| TEXAS INSTRUMENTS INCORPORATED
| Standard Linear and Logic Group
| IBIS Model of SN74AVC32T245
| 32-Bit Dual-Supply Bus Transeiver with Configurable Voltage Translation and
| 3-State Outputs
| This file contains package information for the following:
|  LFBGA 96-pin (GKE)  package as [Component] AVC32T245_GKE
|  LFBGA 96-pin (ZKE)  package as [Component] AVC32T245_ZKE
| This device can be powered at the following Vccs:
|  1.2 volt Vcc
|  1.5 volt Vcc
|  1.8 volt Vcc
|  2.5 volt Vcc
|  3.3 volt Vcc
| This file provides unique models under the [Model Selector] for each Vcc.
| For operation at a specific Vcc, select the appropriate model after each
| [Model Selector] keyword.
[IBIS Ver]   3.2
[Comment char]  |_char
[File Name]   sn74avc32t245.ibs
[File Rev]   1.1 | x_die
[Date]   July 17, 2004
[Source]   Data created from TI-SPICE simulations at TI-SLL.
[Notes]   The following is an IBIS list for the AVC32T245.
   Please contact sllibis@ti.com with questions and
   comments concerning SLL IBIS models.
   - FILE REV HISTORY
   - 1.1 Release IBIS file on 07/17/04
   - This IBIS model was created from the AVC16T245
   - Power clamp data deleted as there is no power-clamp diode.
   - Due to the fact that the Device is 4.6-V Input/Output
   tolarent, the I/O models has some Non-Monotonic Warnings.
[Disclaimer] Property of Texas Instruments Incorporated.  Unauthorized
   reproduction and/or distribution is strictly prohibited.
   This product is protected under copyright law.
   Created  2003, (C) Copyright  2003, Texas Instruments
   Incorporated, All Rights Reserved
   UNLESS THERE IS A SIGNED, WRITTEN AGREEMENT TO THE
   CONTRARY, TEXAS INSTRUMENTS (TI) IS PROVIDING THE IBIS
   MODELS  AND WITHOUT ANY WARRANTY, EXPRESSED OR
   IMPLIED.  TI assumes no liability for:
   1) the accuracy of the IBIS models provided to your
   company;
   2) the proper functioning of these IBIS Models in your
   design or for any resulting applications; or
   3) infringement of patents, copyrights or intellectual
   property rights resulting from your use of these IBIS
   models.
   TI provides IBIS Models as a service to our customers.
   You and your company shall not distribute, sell or give
   these models to anyone else without prior written
   permission from TI.
   TI reserves the right to make changes to our products or
   to discontinue any semiconductor product or service
   without notice, and advises our customers to obtain the
   latest version of relevant information to verify, before
   placing orders, that the information being relied on is
   current.
   Please be aware that your receipt and use of the IBIS
   information provided shall serve as acceptance of these
   terms and conditions.  If you do not accept these terms,
   you should return or destroy the IBIS models and any
   other accompanying information immediately.
| Component AVC32T245_GKE 96-pin LFBGA
[Component]   AVC32T245_GKE
[Manufacturer]  Texas Instruments, Inc.
[Package]
|   typ   min   max
R_pkg   6.700e-02   5.600e-02   8.700e-02
L_pkg   2.067e-09   1.596e-09   2.867e-09
C_pkg   1.810e-13   1.460e-13   2.440e-13
[Pin]   signal_name   model_name   R_pin   L_pin   C_pin
A3   1DIR   AVC32T245_DIR   8.400e-02   2.866e-09   2.140e-13
A2   1B1   AVC32T245_IO   5.600e-02   1.650e-09   1.470e-13
A1   1B2   AVC32T245_IO   5.900e-02   1.761e-09   1.550e-13
B3   GND   GND   8.300e-02   2.828e-09   2.340e-13
B2   1B3   AVC32T245_IO   6.000e-02   1.737e-09   1.570e-13
B1   1B4   AVC32T245_IO   6.100e-02   1.767e-09   1.580e-13
C3   VCCB   POWER   8.100e-02   2.750e-09   2.280e-13
C2   1B5   AVC32T245_IO   5.700e-02   1.664e-09   1.540e-13
C1   1B6   AVC32T245_IO   6.100e-02   1.746e-09   1.620e-13
D3   GND   GND   7.900e-02   2.660e-09   2.390e-13
D2   1B7   AVC32T245_IO   5.600e-02   1.619e-09   1.520e-13
D1   1B8   AVC32T245_IO   6.100e-02   1.703e-09   1.510e-13
E2   2B1   AVC32T245_IO   6.400e-02   1.911e-09   1.680e-13
E1   2B2   AVC32T245_IO   6.100e-02   1.732e-09   1.540e-13
E3   GND   GND   7.900e-02   2.626e-09   2.290e-13
F2   2B3   AVC32T245_IO   6.400e-02   1.862e-09   1.750e-13
F1   2B4   AVC32T245_IO   6.100e-02   1.697e-09   1.520e-13
F3   VCCB   POWER   8.000e-02   2.671e-09   2.320e-13
G2   2B5   AVC32T245_IO   6.500e-02   1.908e-09   1.770e-13
G1   2B6   AVC32T245_IO   6.100e-02   1.682e-09   1.510e-13
G3   GND   GND   8.000e-02   2.678e-09   2.150e-13
H1   2B8   AVC32T245_IO   6.100e-02   1.720e-09   1.590e-13
H2   2B7   AVC32T245_IO   5.600e-02   1.596e-09   1.500e-13
H3   2DIR   AVC32T245_DIR   8.600e-02   2.851e-09   2.440e-13
J3   3DIR   AVC32T245_DIR   8.700e-02   2.852e-09   2.440e-13
J2   3B1   AVC32T245_IO   5.600e-02   1.596e-09   1.500e-13
J1   3B2   AVC32T245_IO   6.200e-02   1.721e-09   1.580e-13
K3   GND   GND   8.000e-02   2.678e-09   2.170e-13
K2   3B3   AVC32T245_IO   6.200e-02   1.741e-09   1.560e-13
K1   3B4   AVC32T245_IO   6.000e-02   1.696e-09   1.580e-13
L3   VCCB   POWER   8.000e-02   2.675e-09   2.200e-13
L2   3B5   AVC32T245_IO   6.100e-02   1.754e-09   1.570e-13
L1   3B6   AVC32T245_IO   6.100e-02   1.702e-09   1.610e-13
M3   GND   GND   7.800e-02   2.628e-09   2.210e-13
M2   3B7   AVC32T245_IO   6.200e-02   1.791e-09   1.580e-13
M1   3B8   AVC32T245_IO   6.100e-02   1.748e-09   1.570e-13
N2   4B1   AVC32T245_IO   6.200e-02   1.762e-09   1.560e-13
N1   4B2   AVC32T245_IO   7.500e-02   2.597e-09   2.180e-13
N3   GND   GND   5.900e-02   1.680e-09   1.610e-13
P2   4B3   AVC32T245_IO   6.200e-02   1.805e-09   1.660e-13
P1   4B4   AVC32T245_IO   5.700e-02   1.661e-09   1.530e-13
P3   VCCB   POWER   8.100e-02   2.751e-09   2.270e-13
R2   4B5   AVC32T245_IO   6.200e-02   1.838e-09   1.630e-13
R1   4B6   AVC32T245_IO   6.300e-02   1.845e-09   1.650e-13
R3   GND   GND   8.300e-02   2.828e-09   2.330e-13
T1   4B7   AVC32T245_IO   6.000e-02   1.754e-09   1.550e-13
T2   4B8   AVC32T245_IO   5.600e-02   1.659e-09   1.480e-13
T3   4DIR   AVC32T245_DIR   8.500e-02   2.867e-09   2.160e-13
T4   4NOE   AVC32T245_NOE   8.400e-02   2.866e-09   2.160e-13
T5   4A8   AVC32T245_IO   5.600e-02   1.658e-09   1.480e-13
T6   4A7   AVC32T245_IO   6.000e-02   1.753e-09   1.550e-13
R4   GND   GND   8.300e-02   2.828e-09   2.320e-13
R6   4A6   AVC32T245_IO   5.900e-02   1.707e-09   1.550e-13
R5   4A5   AVC32T245_IO   6.300e-02   1.838e-09   1.640e-13
P4   VCCA   POWER   8.100e-02   2.751e-09   2.270e-13
P6   4A4   AVC32T245_IO   5.700e-02   1.661e-09   1.530e-13
P5   4A3   AVC32T245_IO   6.500e-02   1.946e-09   1.760e-13
N4   GND   GND   8.200e-02   2.804e-09   2.370e-13
N6   4A2   AVC32T245_IO   5.600e-02   1.616e-09   1.500e-13
N5   4A1   AVC32T245_IO   6.200e-02   1.762e-09   1.550e-13
M6   3A8   AVC32T245_IO   6.100e-02   1.748e-09   1.570e-13
M5   3A7   AVC32T245_IO   6.200e-02   1.791e-09   1.580e-13
M4   GND   GND   7.800e-02   2.628e-09   2.210e-13
L6   3A6   AVC32T245_IO   6.000e-02   1.678e-09   1.590e-13
L5   3A5   AVC32T245_IO   6.200e-02   1.755e-09   1.570e-13
L4   VCCA   POWER   8.000e-02   2.674e-09   2.200e-13
K6   3A4   AVC32T245_IO   6.000e-02   1.673e-09   1.560e-13
K5   3A3   AVC32T245_IO   6.100e-02   1.739e-09   1.560e-13
K4   GND   GND   8.000e-02   2.677e-09   2.170e-13
J6   3A2   AVC32T245_IO   6.100e-02   1.720e-09   1.590e-13
J5   3A1   AVC32T245_IO   5.600e-02   1.596e-09   1.500e-13
J4   3NOE   AVC32T245_NOE   8.700e-02   2.852e-09   2.440e-13
H4   2NOE   AVC32T245_NOE   8.700e-02   2.852e-09   2.440e-13
H5   2A7   AVC32T245_IO   5.600e-02   1.596e-09   1.500e-13
H6   2A8   AVC32T245_IO   6.100e-02   1.720e-09   1.590e-13
G4   GND   GND   8.200e-02   2.793e-09   2.220e-13
G5   2A5   AVC32T245_IO   6.100e-02   1.682e-09   1.510e-13
G6   2A6   AVC32T245_IO   6.400e-02   1.907e-09   1.770e-13
F4   VCCA   POWER   8.000e-02   2.670e-09   2.330e-13
F6   2A4   AVC32T245_IO   6.100e-02   1.697e-09   1.520e-13
F5   2A3   AVC32T245_IO   6.400e-02   1.862e-09   1.750e-13
E4   GND   GND   7.800e-02   2.626e-09   2.300e-13
E6   2A2   AVC32T245_IO   6.100e-02   1.714e-09   1.530e-13
E5   2A1   AVC32T245_IO   6.400e-02   1.911e-09   1.680e-13
D6   1A8   AVC32T245_IO   6.100e-02   1.736e-09   1.530e-13
D5   1A7   AVC32T245_IO   5.600e-02   1.619e-09   1.520e-13
D4   GND   GND   7.900e-02   2.660e-09   2.400e-13
C6   1A6   AVC32T245_IO   5.800e-02   1.629e-09   1.550e-13
C5   1A5   AVC32T245_IO   5.700e-02   1.664e-09   1.540e-13
C4   VCCA   POWER   8.100e-02   2.750e-09   2.280e-13
B6   1A4   AVC32T245_IO   5.900e-02   1.667e-09   1.520e-13
B5   1A3   AVC32T245_IO   5.900e-02   1.736e-09   1.570e-13
B4   GND   GND   8.300e-02   2.827e-09   2.340e-13
A6   1A2   AVC32T245_IO   5.700e-02   1.610e-09   1.460e-13
A5   1A1   AVC32T245_IO   5.600e-02   1.649e-09   1.470e-13
A4   1NOE   AVC32T245_NOE   8.500e-02   2.867e-09   2.140e-13
| Component AVC32T245_ZKE 96-pin LFBGA
[Component]   AVC32T245_ZKE
[Manufacturer]  Texas Instruments, Inc.
[Package]
|   typ   min   max
R_pkg   6.700e-02   5.600e-02   8.700e-02
L_pkg   2.067e-09   1.596e-09   2.867e-09
C_pkg   1.810e-13   1.460e-13   2.440e-13
[Pin]   signal_name   model_name   R_pin   L_pin   C_pin
A3   1DIR   AVC32T245_DIR   8.400e-02   2.866e-09   2.140e-13
A2   1B1   AVC32T245_IO   5.600e-02   1.650e-09   1.470e-13
A1   1B2   AVC32T245_IO   5.900e-02   1.761e-09   1.550e-13
B3   GND   GND   8.300e-02   2.828e-09   2.340e-13
B2   1B3   AVC32T245_IO   6.000e-02   1.737e-09   1.570e-13
B1   1B4   AVC32T245_IO   6.100e-02   1.767e-09   1.580e-13
C3   VCCB   POWER   8.100e-02   2.750e-09   2.280e-13
C2   1B5   AVC32T245_IO   5.700e-02   1.664e-09   1.540e-13
C1   1B6   AVC32T245_IO   6.100e-02   1.746e-09   1.620e-13
D3   GND   GND   7.900e-02   2.660e-09   2.390e-13
D2   1B7   AVC32T245_IO   5.600e-02   1.619e-09   1.520e-13
D1   1B8   AVC32T245_IO   6.100e-02   1.703e-09   1.510e-13
E2   2B1   AVC32T245_IO   6.400e-02   1.911e-09   1.680e-13
E1   2B2   AVC32T245_IO   6.100e-02   1.732e-09   1.540e-13
E3   GND   GND   7.900e-02   2.626e-09   2.290e-13
F2   2B3   AVC32T245_IO   6.400e-02   1.862e-09   1.750e-13
F1   2B4   AVC32T245_IO   6.100e-02   1.697e-09   1.520e-13
F3   VCCB   POWER   8.000e-02   2.671e-09   2.320e-13
G2   2B5   AVC32T245_IO   6.500e-02   1.908e-09   1.770e-13
G1   2B6   AVC32T245_IO   6.100e-02   1.682e-09   1.510e-13
G3   GND   GND   8.000e-02   2.678e-09   2.150e-13
H1   2B8   AVC32T245_IO   6.100e-02   1.720e-09   1.590e-13
H2   2B7   AVC32T245_IO   5.600e-02   1.596e-09   1.500e-13
H3   2DIR   AVC32T245_DIR   8.600e-02   2.851e-09   2.440e-13
J3   3DIR   AVC32T245_DIR   8.700e-02   2.852e-09   2.440e-13
J2   3B1   AVC32T245_IO   5.600e-02   1.596e-09   1.500e-13
J1   3B2   AVC32T245_IO   6.200e-02   1.721e-09   1.580e-13
K3   GND   GND   8.000e-02   2.678e-09   2.170e-13
K2   3B3   AVC32T245_IO   6.200e-02   1.741e-09   1.560e-13
K1   3B4   AVC32T245_IO   6.000e-02   1.696e-09   1.580e-13
L3   VCCB   POWER   8.000e-02   2.675e-09   2.200e-13
L2   3B5   AVC32T245_IO   6.100e-02   1.754e-09   1.570e-13
L1   3B6   AVC32T245_IO   6.100e-02   1.702e-09   1.610e-13
M3   GND   GND   7.800e-02   2.628e-09   2.210e-13
M2   3B7   AVC32T245_IO   6.200e-02   1.791e-09   1.580e-13
M1   3B8   AVC32T245_IO   6.100e-02   1.748e-09   1.570e-13
N2   4B1   AVC32T245_IO   6.200e-02   1.762e-09   1.560e-13
N1   4B2   AVC32T245_IO   7.500e-02   2.597e-09   2.180e-13
N3   GND   GND   5.900e-02   1.680e-09   1.610e-13
P2   4B3   AVC32T245_IO   6.200e-02   1.805e-09   1.660e-13
P1   4B4   AVC32T245_IO   5.700e-02   1.661e-09   1.530e-13
P3   VCCB   POWER   8.100e-02   2.751e-09   2.270e-13
R2   4B5   AVC32T245_IO   6.200e-02   1.838e-09   1.630e-13
R1   4B6   AVC32T245_IO   6.300e-02   1.845e-09   1.650e-13
R3   GND   GND   8.300e-02   2.828e-09   2.330e-13
T1   4B7   AVC32T245_IO   6.000e-02   1.754e-09   1.550e-13
T2   4B8   AVC32T245_IO   5.600e-02   1.659e-09   1.480e-13
T3   4DIR   AVC32T245_DIR   8.500e-02   2.867e-09   2.160e-13
T4   4NOE   AVC32T245_NOE   8.400e-02   2.866e-09   2.160e-13
T5   4A8   AVC32T245_IO   5.600e-02   1.658e-09   1.480e-13
T6   4A7   AVC32T245_IO   6.000e-02   1.753e-09   1.550e-13
R4   GND   GND   8.300e-02   2.828e-09   2.320e-13
R6   4A6   AVC32T245_IO   5.900e-02   1.707e-09   1.550e-13
R5   4A5   AVC32T245_IO   6.300e-02   1.838e-09   1.640e-13
P4   VCCA   POWER   8.100e-02   2.751e-09   2.270e-13
P6   4A4   AVC32T245_IO   5.700e-02   1.661e-09   1.530e-13
P5   4A3   AVC32T245_IO   6.500e-02   1.946e-09   1.760e-13
N4   GND   GND   8.200e-02   2.804e-09   2.370e-13
N6   4A2   AVC32T245_IO   5.600e-02   1.616e-09   1.500e-13
N5   4A1   AVC32T245_IO   6.200e-02   1.762e-09   1.550e-13
M6   3A8   AVC32T245_IO   6.100e-02   1.748e-09   1.570e-13
M5   3A7   AVC32T245_IO   6.200e-02   1.791e-09   1.580e-13
M4   GND   GND   7.800e-02   2.628e-09   2.210e-13
L6   3A6   AVC32T245_IO   6.000e-02   1.678e-09   1.590e-13
L5   3A5   AVC32T245_IO   6.200e-02   1.755e-09   1.570e-13
L4   VCCA   POWER   8.000e-02   2.674e-09   2.200e-13
K6   3A4   AVC32T245_IO   6.000e-02   1.673e-09   1.560e-13
K5   3A3   AVC32T245_IO   6.100e-02   1.739e-09   1.560e-13
K4   GND   GND   8.000e-02   2.677e-09   2.170e-13
J6   3A2   AVC32T245_IO   6.100e-02   1.720e-09   1.590e-13
J5   3A1   AVC32T245_IO   5.600e-02   1.596e-09   1.500e-13
J4   3NOE   AVC32T245_NOE   8.700e-02   2.852e-09   2.440e-13
H4   2NOE   AVC32T245_NOE   8.700e-02   2.852e-09   2.440e-13
H5   2A7   AVC32T245_IO   5.600e-02   1.596e-09   1.500e-13
H6   2A8   AVC32T245_IO   6.100e-02   1.720e-09   1.590e-13
G4   GND   GND   8.200e-02   2.793e-09   2.220e-13
G5   2A5   AVC32T245_IO   6.100e-02   1.682e-09   1.510e-13
G6   2A6   AVC32T245_IO   6.400e-02   1.907e-09   1.770e-13
F4   VCCA   POWER   8.000e-02   2.670e-09   2.330e-13
F6   2A4   AVC32T245_IO   6.100e-02   1.697e-09   1.520e-13
F5   2A3   AVC32T245_IO   6.400e-02   1.862e-09   1.750e-13
E4   GND   GND   7.800e-02   2.626e-09   2.300e-13
E6   2A2   AVC32T245_IO   6.100e-02   1.714e-09   1.530e-13
E5   2A1   AVC32T245_IO   6.400e-02   1.911e-09   1.680e-13
D6   1A8   AVC32T245_IO   6.100e-02   1.736e-09   1.530e-13
D5   1A7   AVC32T245_IO   5.600e-02   1.619e-09   1.520e-13
D4   GND   GND   7.900e-02   2.660e-09   2.400e-13
C6   1A6   AVC32T245_IO   5.800e-02   1.629e-09   1.550e-13
C5   1A5   AVC32T245_IO   5.700e-02   1.664e-09   1.540e-13
C4   VCCA   POWER   8.100e-02   2.750e-09   2.280e-13
B6   1A4   AVC32T245_IO   5.900e-02   1.667e-09   1.520e-13
B5   1A3   AVC32T245_IO   5.900e-02   1.736e-09   1.570e-13
B4   GND   GND   8.300e-02   2.827e-09   2.340e-13
A6   1A2   AVC32T245_IO   5.700e-02   1.610e-09   1.460e-13
A5   1A1   AVC32T245_IO   5.600e-02   1.649e-09   1.470e-13
A4   1NOE   AVC32T245_NOE   8.500e-02   2.867e-09   2.140e-13
| Model AVC32T245_NOE
[Model Selector]   AVC32T245_NOE
AVC32T245_NOE_12   1.2 volt Vcc
AVC32T245_NOE_15   1.5 volt Vcc
AVC32T245_NOE_18   1.8 volt Vcc
AVC32T245_NOE_25   2.5 volt Vcc
AVC32T245_NOE_33   3.3 volt Vcc
| Model AVC32T245_DIR
[Model Selector]   AVC32T245_DIR
AVC32T245_DIR_12   1.2 volt Vcc
AVC32T245_DIR_15   1.5 volt Vcc
AVC32T245_DIR_18   1.8 volt Vcc
AVC32T245_DIR_25   2.5 volt Vcc
AVC32T245_DIR_33   3.3 volt Vcc
| Model AVC32T245_IO
[Model Selector]   AVC32T245_IO
AVC32T245_IO_12   1.2 volt Vcc
AVC32T245_IO_15   1.5 volt Vcc
AVC32T245_IO_18   1.8 volt Vcc
AVC32T245_IO_25   2.5 volt Vcc
AVC32T245_IO_33   3.3 volt Vcc
| Models and submodels in the file (15): AVC32T245_NOE_12 (Input), AVC32T245_NOE_15 (Input), AVC32T245_NOE_18 (Input), AVC32T245_NOE_25 (Input), AVC32T245_NOE_33 (Input), AVC32T245_DIR_12 (Input), AVC32T245_DIR_15 (Input), AVC32T245_DIR_18 (Input), AVC32T245_DIR_25 (Input), AVC32T245_DIR_33 (Input), AVC32T245_IO_12 (I/O), AVC32T245_IO_15 (I/O), AVC32T245_IO_18 (I/O), AVC32T245_IO_25 (I/O), AVC32T245_IO_33 (I/O)
